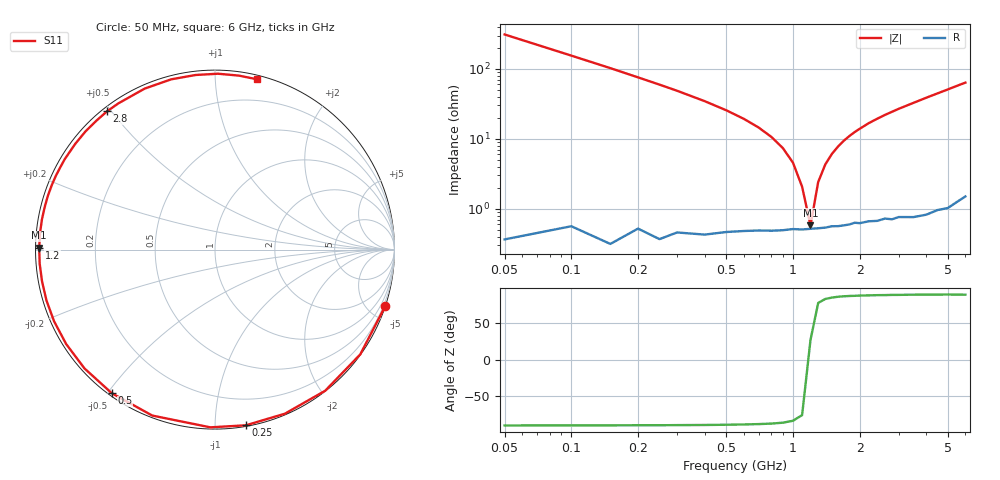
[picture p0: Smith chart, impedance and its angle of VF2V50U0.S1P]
! Infineon Technologies  Discrete & RF Semiconductors
! BBY 58-03
! Si Tuning Diode in SOD323
! VR = 2.5 V
! S-Parameters:  June  1999
# GHz  S  MA  R  50
!  f  S11
! GHz  MAG  ANG
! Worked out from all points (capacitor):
!   34 points, 50 MHz to 6 GHz, reference 50 ohm
!   read as one part to ground: C = 10.2 pF near 50 MHz
!   lowest |Z| = 581 mohm at 1.2 GHz (marker M1)
!   series resonance near 1.188 GHz, so ESL is about 1.8 nH
!   S11 on the Smith chart (normalised r, x): 50 MHz: 0.01, -6.21; 250 MHz: 0.01, -1.19; 500 MHz: 0.01, -0.51; 1.2 GHz: 0.01, +0.01; 2.8 GHz: 0.01, +0.49; 6 GHz: 0.03, +1.27
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0.05  0.9996 -18.3
0.1  0.9979 -35.8
0.15  0.9976 -52.0
0.2  0.9937 -66.9
0.25  0.9939 -80.0
0.3  0.9906 -91.5
0.4  0.9885 -110.7
0.5  0.9853 -125.7
0.6  0.9834 -137.7
0.7  0.9821 -147.6
0.8  0.9815 -156.0
0.9  0.9808 -163.2
1  0.9798 -169.6
1.1  0.9799 -175.4
1.2  0.9795 179.4
1.4  0.9788 170.2
1.6  0.9781 162.3
1.9  0.9765 151.9
2.2  0.9764 142.9
2.4  0.9769 137.6
2.8  0.9773 128.0
3  0.9766 123.5
3.5  0.9789 113.6
4  0.9796 104.4
4.5  0.9789 96.3
5  0.98 89.0
5.5  0.9785 82.2
6  0.9773 76.3
